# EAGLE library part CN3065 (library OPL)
USB-Compatible Lithiumt-Ion Battery Charger with Thermal Regulation http://www.consonance-elec.com/pdf/%E6%8A%80%E6%9C%AF%E8%AF%B4%E6%98%8E%E4%B9%A6/DSC-CN3065.pdf
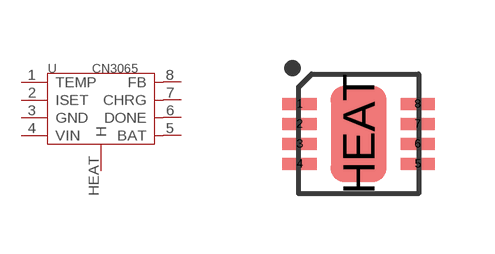
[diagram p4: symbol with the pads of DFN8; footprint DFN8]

Designator prefix U

## CN3065-1320040P1  [DFN8]
1  TEMP  in
2  ISET
3  GND  sup
4  VIN  in
5  BAT
6  DONE
7  CHRG
8  FB  in
HEAT  H

## Footprint DFN8 (pad centres in mm)
smd 0.854 x 0.3: 1 -1.477,0.75; 2 -1.477,0.25; 3 -1.477,-0.25; 4 -1.477,-0.75; 5 1.477,-0.75; 6 1.477,-0.25; 7 1.477,0.25; 8 1.477,0.75
smd 1.397 x 2.413: HEAT 0,0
